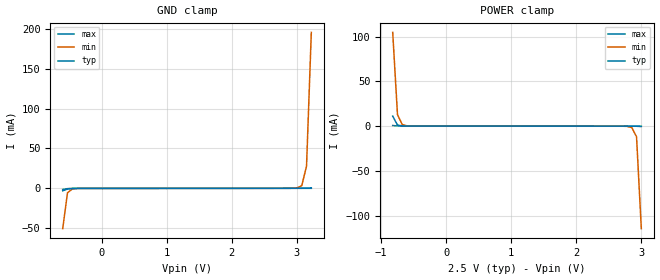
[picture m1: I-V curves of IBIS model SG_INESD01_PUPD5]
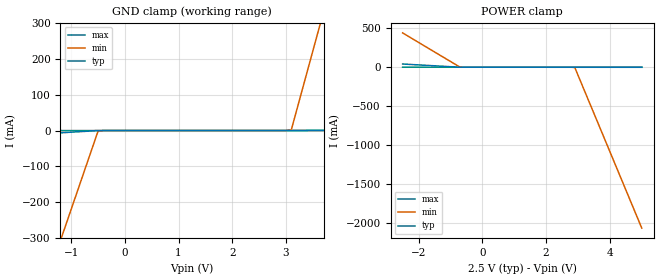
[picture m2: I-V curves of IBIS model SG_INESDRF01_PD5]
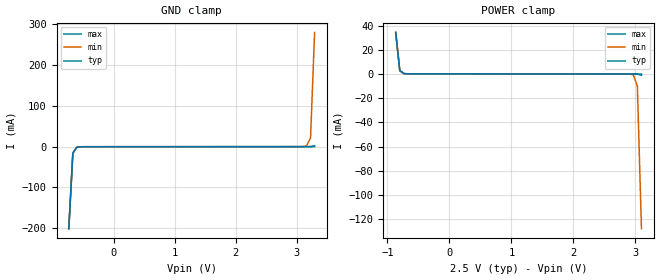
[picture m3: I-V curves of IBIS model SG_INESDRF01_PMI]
|   This file is an IBIS representation of the   |
|   Integrated Device Technology Inc   |
|   IDTSLVD1204I   |
|   1:4 LVDS OUTPUT FANOUT BUFFER   |
[IBIS Ver]   4.1
[File name]   8slvd1204i.ibs
[File Rev]   1.0
[Date]   25 Feb 2013
[Source]   Originated at Integrated Device Technology, Inc.
[Disclaimer]
IDT hereby grants the user of this IBIS model a non-exclusive,
nontransferable license to use this IBIS model under the following terms.
Before using this IBIS model, the user should read this license.
If the user does not accept these terms,  the IBIS model should be
returned to IDT within 30 days.
   The user is granted this license only to use the IBIS model and
is not granted rights to sell, load, rent, lease or license the IBIS
model in whole or in part, or in modified form to anyone other than
user. User may modify the IBIS model to suit its specific
applications but rights to derivative works and such modifications
shall belong to IDT.
   This IBIS model is provided on an "AS IS" basis and IDT makes
absolutely no warranty with respect to the information contained
herein. IDT DISCLAIMS AND CUSTOMER WAIVES ALL WARRANTIES, EXPRESS
OR IMPLIED, INCLUDING WARRANTIES OF MERCHANTABILITY OR FITNESS FOR
A PARTICULAR PURPOSE. The entire risk as to quality and performance
is with the Customer. ACCORDINGLY, IN NO EVENT SHALL THE COMPANY BE
LIABLE FOR ANY DAMAGES, WHETHER IN CONTRACT OR TORT,INCLUDING ANY
LOST PROFITS OR OTHER INCIDENTAL, CONSEQUENTIAL, EXEMPLARY, OR
PUNITIVE DAMAGES ARISING OUT OF THE USE OR APPLICATION OF THE IBIS
model provided in this package. Further, IDT reserves the right to
make changes without notice to any product herein to improve
reliability, function, or design. IDT does not convey any license
under patent rights or any other intellectual property rights,
including those of third parties.
   IDT is not obligated to provide maintenance or support
for the licensed IBIS model.
[Copyright] Copyright 2012 by Integrated Device Technology, Inc.
[Component]   IDT8SLVP1204NLGI
[Manufacturer] Integrated Device Technology, Inc.
[Package]
|QFN 16
|lead + wire   typ   min   max
R_pkg   72.4655m   58.886m   86.045m
L_pkg   1.47175nH   1.11650nH   1.77850n
C_pkg   0.07747pF   0.07444pF   0.08050pF
[Pin] signal_name  model_name   R_pin   L_pin   C_pin
1   VEE   GND   86.045m   1.77850nH   0.08050pF
2   SEL   SG_INESD01_PUPD5   58.886m   1.11650nH   0.07444pF
3   PCLK1   SG_INESDRF01_PD5   58.886m   1.11650nH   0.07444pF
4   nPCLK1   SG_INESDRF01_PMI   86.045m   1.77850nH   0.08050pF
5   VCC   POWER   86.045m   1.77850nH   0.08050pF
6   PCLK0   SG_INESDRF01_PD5   58.886m   1.11650nH   0.07444pF
7   nPCLK0   SG_INESDRF01_PMI   58.886m   1.11650nH   0.07444pF
8   VREF   NC   86.045m   1.77850nH   0.08050pF
9   Q0   SG_OPECL_LVDS03_   86.045m   1.77850nH   0.08050pF
10   nQ0   SG_OPECL_LVDS03_   58.886m   1.11650nH   0.07444pF
11   Q1   SG_OPECL_LVDS03_   58.886m   1.11650nH   0.07444pF
12   nQ1   SG_OPECL_LVDS03_   86.045m   1.77850nH   0.08050pF
13   Q2   SG_OPECL_LVDS03_   86.045m   1.77850nH   0.08050pF
14   nQ2   SG_OPECL_LVDS03_   58.886m   1.11650nH   0.07444pF
15   Q3   SG_OPECL_LVDS03_   58.886m   1.11650nH   0.07444pF
16   nQ3   SG_OPECL_LVDS03_   86.045m   1.77850nH   0.08050pF
[Diff Pin]  inv_pin   vdiff   tdelay_typ   tdelay_min   tdelay_max
3   4   0.2   NA   NA   NA
6   7   0.2   NA   NA   NA
9   10   NA   0   0   0
11   12   NA   0   0   0
13   14   NA   0   0   0
15   16   NA   0   0   0
| Models and submodels in the file (4): SG_INESD01_PUPD5 (Input), SG_INESDRF01_PD5 (Input), SG_INESDRF01_PMI (Input), SG_OPECL_LVDS03_ (Output)
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[Model]   SG_INESD01_PUPD5
Model_type   Input
Polarity   Non-Inverting
Vinl = 0.7V
Vinh = 1.7V
|   typ   min   max
C_comp   2pF   1.5pF   2.5pF
|   typ   min   max
[Voltage range]   2.5V   2.375V   2.625V
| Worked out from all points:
|   GND clamp passes 1 mA (typ) near -0.53 V on its own axis
|   POWER clamp passes 1 mA (typ) near -0.74 V on its own axis
[GND_clamp]
|Voltage   I (typ)   I (min)   I (max)
|Note, modeling breaks down at 250mA and above.  This is well beyond the functional   |
|operating range of the device.  Should this scenario occur, catastrophic failure and   |
|possible damage to the device and/or board is of higher concern than the I-V curve   |
|behavior.  The IBIS checker will flag currents in excess of 10A with warnings.  Lines   |
|with currents in excess of 0.35 A have been commented out.  The points still remain|
|available to the user if the user desires to use them.   |
|-2.40000e+00   -1.41362e+08   -1.15074e+08   -1.85518e+08
|-2.30000e+00   -1.28615e+08   -1.04462e+08   -1.69217e+08
|-2.20000e+00   -1.15868e+08   -9.38499e+07   -1.52915e+08
|-2.10000e+00   -1.03120e+08   -8.32381e+07   -1.36614e+08
|-2.00000e+00   -9.03731e+07   -7.26263e+07   -1.20313e+08
|-1.99900e+00   -9.02456e+07   -7.25201e+07   -1.20150e+08
|-1.92545e+00   -8.08697e+07   -6.47150e+07   -1.08160e+08
|-1.85190e+00   -7.14938e+07   -5.69098e+07   -9.61705e+07
|-1.77834e+00   -6.21179e+07   -4.91046e+07   -8.41807e+07
|-1.70479e+00   -5.27420e+07   -4.12994e+07   -7.21909e+07
|-1.63124e+00   -4.33661e+07   -3.34943e+07   -6.02010e+07
|-1.55769e+00   -3.39902e+07   -2.56891e+07   -4.82112e+07
|-1.48414e+00   -2.46143e+07   -1.78839e+07   -3.62214e+07
|-1.41059e+00   -1.52384e+07   -1.00787e+07   -2.42316e+07
|-1.33703e+00   -5.94947e+06   -4.08072e+06   -1.22418e+07
|-1.26348e+00   -2.71387e+06   -2.47508e+06   -3.36864e+06
|-1.18993e+00   -1.45881e+06   -1.46918e+06   -1.51358e+06
|-1.11638e+00   -3.24411e+05   -5.18604e+05   -1.66319e+05
|-1.04283e+00   -1.85381e+04   -4.97628e+04   -4.28573e+03
|-9.69276e-01   -1.06576e+03   -4.59957e+03   -1.15147e+02
|-8.95724e-01   -6.50258e+01   -4.30083e+02   -4.30239e+00
|-8.22172e-01   -5.12565e+00   -4.32219e+01   -1.23773e-01
|-7.48621e-01   -3.14355e-01   -5.32330e+00   -9.48978e-03
|-6.75069e-01   -2.16093e-02   -5.24003e-01   -3.59262e-03
-601.5mV  -3.047mA   -50.49mA   -1.385mA
-528mV    -811.3uA   -5.614mA   -336uA
-454.4mV  -205.9uA   -820.9uA   -90.77uA
2.929V    66.32uA    167.4uA    59.73uA
3.003V    71.29uA    575.2uA    62.44uA
3.076V    89.08uA    3.284mA    65.17uA
3.15V     179.3uA    27.92mA    67.96uA
3.223V    637.3uA    195.4mA    71.81uA
| 3.29672e+00   4.67377e-03   1.45088e+00   8.64327e-05
| 3.37028e+00   6.37395e-02   1.35768e+01   1.74735e-04
| 3.44383e+00   7.33950e-01   1.27134e+02   6.54087e-04
| 3.51738e+00   1.08087e+01   1.33404e+03   7.79842e-03
| 3.59093e+00   1.59019e+02   1.43927e+04   2.39972e-01
| 3.66448e+00   2.70591e+03   1.55924e+05   7.54089e+00
| 3.73803e+00   4.72566e+04   1.69009e+06   2.37047e+02
| 3.81159e+00   8.27346e+05   8.20594e+06   9.02257e+03
| 3.88514e+00   7.53030e+06   1.50662e+07   3.50631e+05
| 3.95869e+00   1.57711e+07   2.19264e+07   7.35650e+06
| 4.03224e+00   2.40119e+07   2.87866e+07   1.78947e+07
| 4.10579e+00   3.22527e+07   3.56469e+07   2.84330e+07
| 4.17934e+00   4.04934e+07   4.25071e+07   3.89712e+07
| 4.25290e+00   4.87342e+07   4.93673e+07   4.95095e+07
| 4.32645e+00   5.69750e+07   5.62275e+07   6.00477e+07
| 4.40000e+00   6.52158e+07   6.30878e+07   7.05859e+07
| 4.40100e+00   6.53278e+07   6.31810e+07   7.07292e+07
| 4.52080e+00   7.87503e+07   7.43549e+07   8.78937e+07
| 4.64060e+00   9.21728e+07   8.55287e+07   1.05058e+08
| 4.76040e+00   1.05595e+08   9.67026e+07   1.22223e+08
| 4.88020e+00   1.19018e+08   1.07876e+08   1.39387e+08
| 5.00000e+00   1.32440e+08   1.19050e+08   1.56552e+08
[Power_clamp]
|Voltage   I (typ)   I (min)   I (max)
|Note, modeling breaks down at 250mA and above.  This is well beyond the functional   |
|operating range of the device.  Should this scenario occur, catastrophic failure and   |
|possible damage to the device and/or board is of higher concern than the I-V curve   |
|behavior.  The IBIS checker will flag currents in excess of 10A with warnings.  Lines   |
|with currents in excess of 0.35 A have been commented out.  The points still remain|
|available to the user if the user desires to use them.   |
|-2.40000e+00   1.21236e+08   9.80643e+07   1.60134e+08
|-2.30000e+00   1.10032e+08   8.87372e+07   1.45806e+08
|-2.20000e+00   9.88280e+07   7.94101e+07   1.31478e+08
|-2.10000e+00   8.76239e+07   7.00831e+07   1.17151e+08
|-2.00000e+00   7.64199e+07   6.07560e+07   1.02823e+08
|-1.99900e+00   7.63078e+07   6.06627e+07   1.02680e+08
|-1.92545e+00   6.80670e+07   5.38025e+07   9.21417e+07
|-1.85190e+00   5.98263e+07   4.69423e+07   8.16034e+07
|-1.77834e+00   5.15855e+07   4.00820e+07   7.10652e+07
|-1.70479e+00   4.33447e+07   3.32218e+07   6.05269e+07
|-1.63124e+00   3.51039e+07   2.63616e+07   4.99887e+07
|-1.55769e+00   2.68631e+07   1.95014e+07   3.94505e+07
|-1.48414e+00   1.86223e+07   1.26411e+07   2.89122e+07
|-1.41059e+00   1.03815e+07   5.78090e+06   1.83740e+07
|-1.33703e+00   2.22772e+06   7.27848e+05   7.83574e+06
|-1.26348e+00   1.27227e+05   6.71549e+04   4.14145e+05
|-1.18993e+00   7.27369e+03   6.20285e+03   1.06555e+04
|-1.11638e+00   4.20825e+02   5.77724e+02   2.79192e+02
|-1.04283e+00   2.67170e+01   5.65791e+01   8.79047e+00
|-9.69276e-01   1.83295e+00   6.28356e+00   2.79050e-01
|-8.95724e-01   1.49870e-01   6.80177e-01   9.03909e-03
-822.2mV  11.17mA    104.6mA    707.2uA
-748.6mV  1.148mA    12.8mA     183.4uA
-675.1mV  262uA      1.673mA    87.93uA
-528mV    74.72uA    123.5uA    68.09uA
2.708V    -57.41uA   -90.07uA   -51.57uA
2.855V    -70.39uA   -1.568mA   -57.01uA
2.929V    -135.2uA   -11.88mA   -59.76uA
3.003V    -509uA     -114.5mA   -63.59uA
| 3.07607e+00   -1.88385e-03   -1.21169e+00   -8.77221e-05
| 3.14962e+00   -9.80201e-03   -1.09449e+01   -3.12408e-04
| 3.22317e+00   -1.19949e-01   -9.57344e+01   -1.31293e-03
| 3.29672e+00   -2.00997e+00   -9.90823e+02   -3.46250e-03
| 3.37028e+00   -2.60228e+01   -1.06686e+04   -8.88627e-03
| 3.44383e+00   -3.99523e+02   -1.15534e+05   -1.06196e-01
| 3.51738e+00   -6.89109e+03   -8.53393e+05   -3.70174e+00
| 3.59093e+00   -1.20491e+05   -1.81140e+06   -9.81142e+01
| 3.66448e+00   -1.06150e+06   -2.89788e+06   -3.62973e+03
| 3.73803e+00   -2.24116e+06   -5.37700e+06   -1.40814e+05
| 3.81159e+00   -4.15636e+06   -1.28378e+07   -1.44593e+06
| 3.88514e+00   -1.19944e+07   -2.06430e+07   -3.23911e+06
| 3.95869e+00   -2.13703e+07   -2.84482e+07   -1.16966e+07
| 4.03224e+00   -3.07462e+07   -3.62533e+07   -2.36864e+07
| 4.10579e+00   -4.01221e+07   -4.40585e+07   -3.56762e+07
| 4.17934e+00   -4.94980e+07   -5.18637e+07   -4.76660e+07
| 4.25290e+00   -5.88739e+07   -5.96689e+07   -5.96558e+07
| 4.32645e+00   -6.82498e+07   -6.74740e+07   -7.16456e+07
| 4.40000e+00   -7.76257e+07   -7.52792e+07   -8.36354e+07
| 4.40100e+00   -7.77532e+07   -7.53853e+07   -8.37984e+07
| 4.52080e+00   -9.30245e+07   -8.80983e+07   -1.03327e+08
| 4.64060e+00   -1.08296e+08   -1.00811e+08   -1.22856e+08
| 4.76040e+00   -1.23567e+08   -1.13524e+08   -1.42385e+08
| 4.88020e+00   -1.38839e+08   -1.26237e+08   -1.61914e+08
| 5.00000e+00   -1.54110e+08   -1.38950e+08   -1.81443e+08
[Model]   SG_INESDRF01_PD5
Model_type   Input
Polarity   Non-Inverting
Vinl = 0.7V
Vinh = 1.7V
|   typ   min   max
C_comp   2pF   1.5pF   2.5pF
|   typ   min   max
[Voltage range]   2.5V   2.375V   2.625V
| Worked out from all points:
|   GND clamp passes 1 mA (typ) near -0.60 V on its own axis
|   POWER clamp passes 1 mA (typ) near -0.74 V on its own axis
[GND_clamp]
|Voltage   I (typ)   I (min)   I (max)
-2.5V     -18.58mA   -877mA     -81.82uA
-1.2V     -6.522mA   -308.1mA   -34.67uA
-1.1V     -5.594mA   -264.4mA   -31.05uA
-500mV    -29.15uA   -1.793mA   -9.284uA
3V        59.28uA    149uA      55.63uA
3.1V      62.21uA    2.306mA    57.48uA
3.6V      307uA      277.5mA    66.76uA
3.7V      355.9uA    332.5mA    68.61uA
5V        992.2uA    1.048A     92.73uA
[Power_clamp]
|Voltage   I (typ)   I (min)   I (max)
-2.5V     41.6mA     441.8mA    990.4uA
-700mV    111.2uA    1.06mA     62uA
2.9V      -8.294uA   -4.02mA    -5.099uA
5V        -446.3uA   -2.07A     -44.04uA
[Model]   SG_INESDRF01_PMI
Model_type   Input
Polarity   Non-Inverting
Vinl = 0.7V
Vinh = 1.7V
|   typ   min   max
C_comp   2pF   1.5pF   2.5pF
|   typ   min   max
[Voltage range]   2.5V   2.375V   2.625V
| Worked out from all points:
|   GND clamp passes 1 mA (typ) near -0.59 V on its own axis
|   POWER clamp passes 1 mA (typ) near -0.75 V on its own axis
[GND_clamp]
|Voltage   I (typ)   I (min)   I (max)
|Note, modeling breaks down at 250mA and above.  This is well beyond the functional   |
|operating range of the device.  Should this scenario occur, catastrophic failure and   |
|possible damage to the device and/or board is of higher concern than the I-V curve   |
|behavior.  The IBIS checker will flag currents in excess of 10A with warnings.  Lines   |
|with currents in excess of 0.35 A have been commented out.  The points still remain|
|available to the user if the user desires to use them.   |
|-2.20000e+00   -1.14988e+08   -1.14988e+08   -1.14988e+08
|-1.90000e+00   -7.70006e+07   -7.70006e+07   -7.70006e+07
|-1.60000e+00   -3.90134e+07   -3.90134e+07   -3.90134e+07
|-1.30000e+00   -3.64698e+06   -3.64698e+06   -3.64698e+06
|-1.00000e+00   -3.68175e+03   -3.68175e+03   -3.68175e+03
|-9.99000e-01   -3.54242e+03   -3.54242e+03   -3.54242e+03
|-9.32920e-01   -2.80614e+02   -2.80614e+02   -2.80614e+02
|-8.66839e-01   -2.48146e+01   -2.48145e+01   -2.48146e+01
|-8.00759e-01   -2.58538e+00   -2.58536e+00   -2.58542e+00
-734.7mV  -201mA     -200.9mA   -201mA
-668.6mV  -15.68mA   -15.66mA   -15.72mA
-602.5mV  -1.286mA   -1.264mA   -1.32mA
3.032V    70.86uA    62.91uA    96.29uA
3.164V    89.5uA     1.748mA    103.8uA
3.23V     252uA      21.83mA    108.8uA
3.296V    2.313mA    280.3mA    128.9uA
| 3.36231e+00   2.87999e-02   3.60620e+00   3.43458e-04
| 3.42839e+00   3.69663e-01   4.00180e+01   3.06146e-03
| 3.49447e+00   4.75655e+00   4.78794e+02   3.79983e-02
| 3.56055e+00   5.20177e+01   6.09553e+03   4.87593e-01
| 3.62663e+00   6.29944e+02   7.83528e+04   6.23482e+00
| 3.69271e+00   8.03755e+03   1.00828e+06   6.77568e+01
| 3.75879e+00   1.03343e+05   7.21319e+06   8.29220e+02
| 3.82487e+00   1.32990e+06   1.45676e+07   1.05990e+04
| 3.89095e+00   8.01015e+06   2.19219e+07   1.36306e+05
| 3.95703e+00   1.53645e+07   2.92763e+07   1.75412e+06
| 4.02311e+00   2.27189e+07   3.66307e+07   8.80712e+06
| 4.08920e+00   3.00733e+07   4.39850e+07   1.61615e+07
| 4.15528e+00   3.74276e+07   5.13394e+07   2.35159e+07
| 4.22136e+00   4.47820e+07   5.86938e+07   3.08702e+07
| 4.28744e+00   5.21364e+07   6.60481e+07   3.82246e+07
| 4.35352e+00   5.94907e+07   7.34025e+07   4.55790e+07
| 4.41960e+00   6.68451e+07   8.07569e+07   5.29333e+07
| 4.48568e+00   7.41995e+07   8.81112e+07   6.02877e+07
| 4.55176e+00   8.15538e+07   9.54656e+07   6.76421e+07
| 4.61784e+00   8.89082e+07   1.02820e+08   7.49964e+07
| 4.68392e+00   9.62626e+07   1.10174e+08   8.23508e+07
| 4.75000e+00   1.03617e+08   1.17529e+08   8.97052e+07
| 4.75100e+00   1.03728e+08   1.17640e+08   8.98165e+07
| 4.80080e+00   1.09271e+08   1.23182e+08   9.53589e+07
| 4.85060e+00   1.14813e+08   1.28725e+08   1.00901e+08
| 4.90040e+00   1.20356e+08   1.34267e+08   1.06444e+08
| 4.95020e+00   1.25898e+08   1.39810e+08   1.11986e+08
| 5.00000e+00   1.31440e+08   1.45352e+08   1.17529e+08
[Power_clamp]
|Voltage   I (typ)   I (min)   I (max)
|Note, modeling breaks down at 250mA and above.  This is well beyond the functional   |
|operating range of the device.  Should this scenario occur, catastrophic failure and   |
|possible damage to the device and/or board is of higher concern than the I-V curve   |
|behavior.  The IBIS checker will flag currents in excess of 10A with warnings.  Lines   |
|with currents in excess of 0.35 A have been commented out.  The points still remain|
|available to the user if the user desires to use them.   |
|-2.20000e+00   9.80522e+07   9.80522e+07   9.80522e+07
|-1.90000e+00   6.46640e+07   6.46640e+07   6.46640e+07
|-1.60000e+00   3.12757e+07   3.12757e+07   3.12757e+07
|-1.30000e+00   5.08353e+05   5.08353e+05   5.08353e+05
|-1.00000e+00   5.86787e+00   5.86785e+00   5.86791e+00
|-9.99000e-01   5.65233e+00   5.65230e+00   5.65237e+00
|-9.32920e-01   4.40386e-01   4.40360e-01   4.40425e-01
-866.8mV  34.3mA     34.27mA    34.33mA
-800.8mV  2.74mA     2.715mA    2.777mA
-734.7mV  285.4uA    261.5uA    321.2uA
2.834V    -62.94uA   -51.69uA   -85.19uA
2.966V    -74.3uA    -822.6uA   -92.64uA
3.032V    -149.9uA   -9.985mA   -96.92uA
3.098V    -1.091mA   -127.9mA   -108.1uA
